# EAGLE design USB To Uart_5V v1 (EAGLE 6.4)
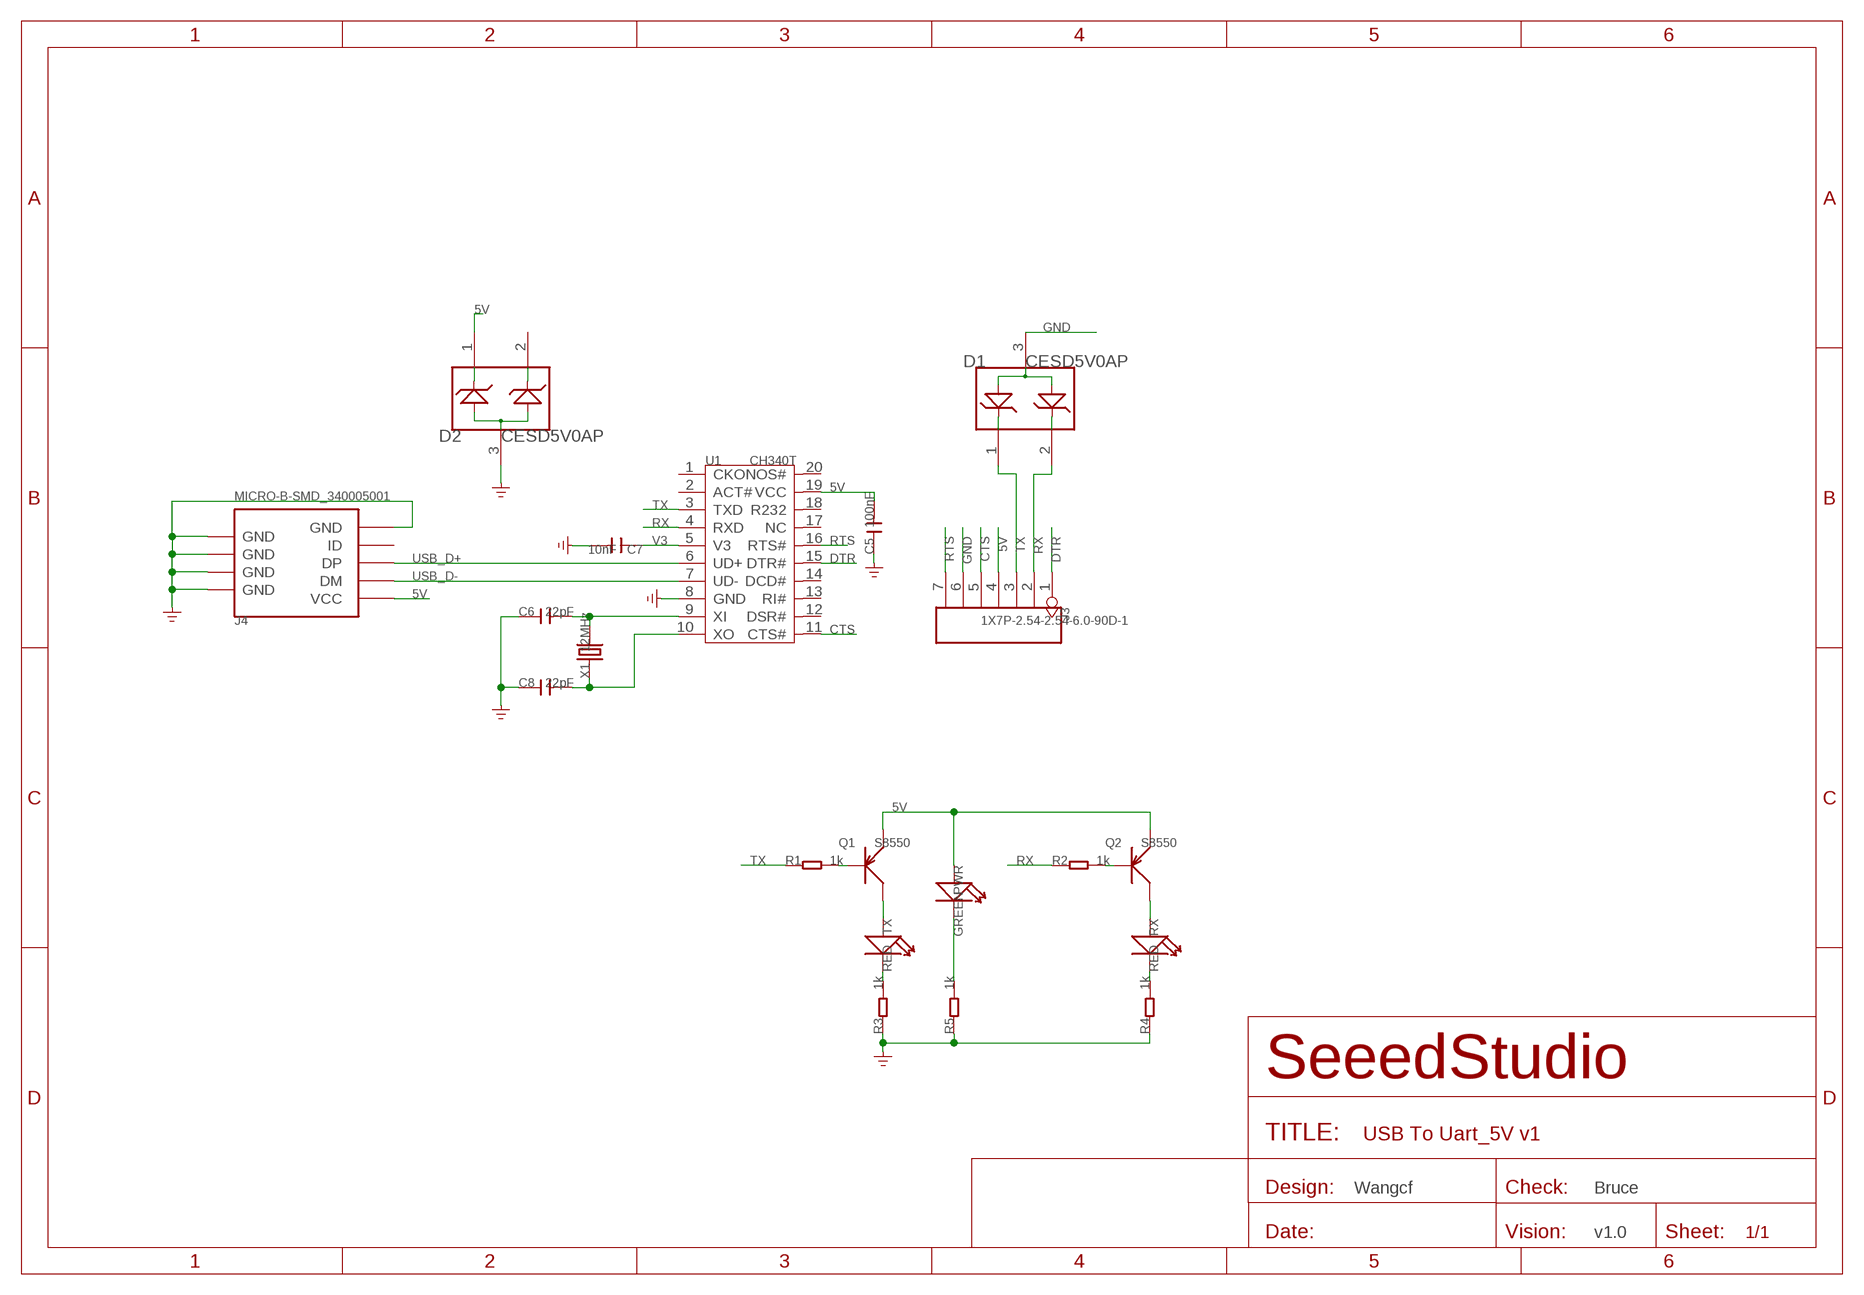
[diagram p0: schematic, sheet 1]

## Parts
C5  100nF  C-0402  [C0402]
C6  22pF  C-0402  [C0402]
C7  10nF  C-0402  [C0402]
C8  22pF  C-0402  [C0402]
D1  CESD5V0AP  D-ESD-3P  [SOT23]
D2  CESD5V0AP  D-ESD-3P  [SOT23]
J3  1X7P-2.54-2.54-6.0-90D-1  HEADER-7P  [7P-2.54-65/35MIL]
J4  MICRO-B-SMD_340005001  USB-MINIUSB-5P-MICRO  [MICRO-USB]
PWR  GREEN  LED'0603'  [LED-0603]
Q1  S8550  TRANSISTOR-PNP-SOT23  [SOT23]
Q2  S8550  TRANSISTOR-PNP-SOT23  [SOT23]
R1  1k  R-0402  [R0402]
R2  1k  R-0402  [R0402]
R3  1k  R-0402  [R0402]
R4  1k  R-0402  [R0402]
R5  1k  R-0402  [R0402]
RX  RED  LED'0603'  [LED-0603]
TX  RED  LED'0603'  [LED-0603]
U1  CH340T  [SSOP20]
X1  12MHz  CRYSTAL'HC49UP'  [HC49UP]

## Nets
5V: C5.2 D2.1 J3.4 J4.1(VCC) PWR.+ Q1.2(E) Q2.2(E) U1.19(VCC)
CTS: J3.5 U1.11(CTS#)
DTR: J3.1 U1.15(DTR#)
GND: C5.1 C6.1 C7.2 C8.1 D1.3 D2.3 J3.6 J4.5(GND) J4.S1(GND) J4.S2(GND) J4.S3(GND) J4.S4(GND) J4.S5(GND) J4.S6(GND) R3.1 R4.1 R5.1 U1.8(GND)
N$1: Q1.3(C) TX.+
N$2: Q2.3(C) RX.+
N$4: C6.2 U1.9(XI) X1.2
N$5: C8.2 U1.10(XO) X1.1
N$6: R3.2 TX.-
N$7: Q1.1(B) R1.2
N$8: Q2.1(B) R2.2
N$10: R4.2 RX.-
N$12: PWR.- R5.2
RTS: J3.7 U1.16(RTS#)
RX: D1.2 J3.2 R2.1 U1.4(RXD)
TX: D1.1 J3.3 R1.1 U1.3(TXD)
USB_D+: J4.3(DP) U1.6(UD+)
USB_D-: J4.2(DM) U1.7(UD-)
V3: C7.1 U1.5(V3)
Unconnected: D2.2 J4.4(ID) U1.1(CKO) U1.2(ACT#) U1.12(DSR#) U1.13(RI#) U1.14(DCD#) U1.17(NC) U1.18(R232) U1.20(NOS#)

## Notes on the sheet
- Wangcf | Bruce
- v1.0

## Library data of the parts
C5-C8 = Discrete:C*: Ceramic Capacitors
D1 D2 = Discrete:D-ESD-3P
J3 = Connector :HEADER-7P
J4 = Connector :USB-MINIUSB-5P
PWR RX TX = Discrete:LED*
Q1 Q2 = Discrete:TRANSISTOR-PNP*: PNP audion
R1-R5 = Discrete:R*
U1 = template:CH340T
X1 = Discrete:CRYSTAL*: CRYSTAL

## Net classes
0 default: width 0.152 mm, drill 0.305 mm, clearance 0.152 mm

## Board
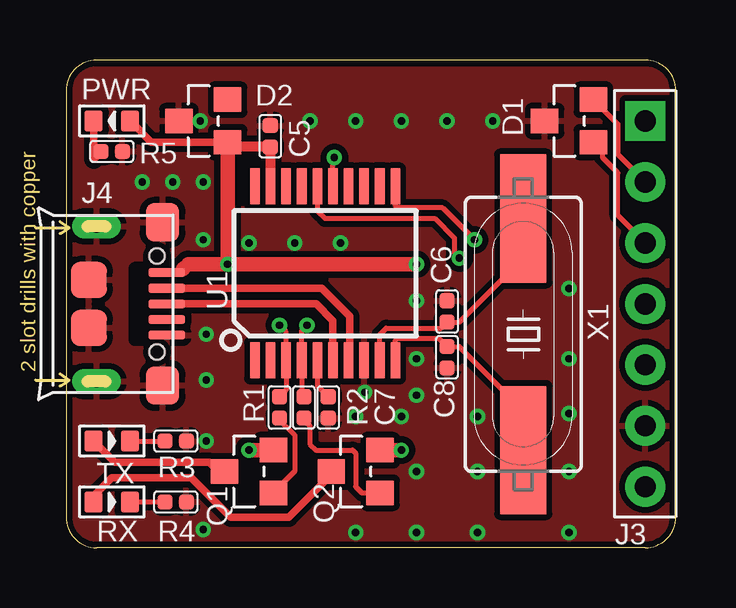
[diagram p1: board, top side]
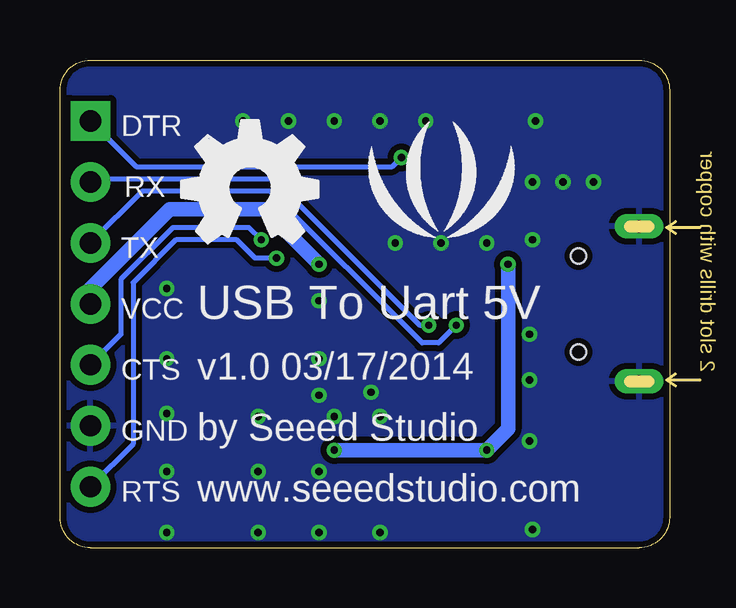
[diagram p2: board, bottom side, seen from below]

Size 25.4 x 20.32 mm. Coordinates in mm from the lower left corner, seen from the top.
Outline: 0,1.27 arc90 1.27,0
Outline: 24.13,0 arc90 25.4,1.27
Outline: 25.4,19.05 arc90 24.13,20.32
Outline: 1.27,20.32 arc90 0,19.05
Outline: 0,1.27 arc90 1.27,0
Outline: 24.13,0 arc90 25.4,1.27
Outline: 25.4,19.05 arc90 24.13,20.32
Outline: 1.27,20.32 arc90 0,19.05
Outline: 0,19.05 0,1.27
Outline: 0,1.27 arc90 1.27,0
Outline: 24.13,0 arc90 25.4,1.27
Outline: 25.4,1.27 25.4,19.05
Outline: 25.4,19.05 arc90 24.13,20.32
Outline: 24.13,20.32 1.27,20.32
Outline: 1.27,20.32 arc90 0,19.05
Outline: 24.13,0 1.27,0
Copper layers (1*16): Top 0.035mm / dielectric 1.5mm / Bottom 0.035mm
Design rules "SeeedStudio_2layer_DRU_no_angle_20140221 *": minimum track width 6mil, minimum drill 12mil, track to track 6mil, track to pad 6mil, pad to pad 6mil, via to via 6mil, smd to smd 0mil, copper to edge 10mil, drill to drill 10mil, minimum pad ring 10mil, minimum via ring 6mil, stop-mask expansion 2mil, vias tented up to drill 25mil, thermal gap 10mil

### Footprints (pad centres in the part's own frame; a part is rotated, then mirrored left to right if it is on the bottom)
C0402 = smd 0.635 x 0.635: 1 -0.445,0; 2 0.445,0
SOT23 = smd 1.016 x 1.143: 1 -0.889,-1.016; 2 0.889,-1.016; 3 0,1.016
7P-2.54-65/35MIL = drill 0.889 pad 1.651 square: 1 0,7.62 | drill 0.889 pad 1.651: 2 0,5.08; 3 0,2.54; 4 0,0; 5 0,-2.54; 6 0,-5.08; 7 0,-7.62
MICRO-USB = smd 0.381 x 1.524: 1 -1.3,-0.25; 2 -0.65,-0.25; 3 0,-0.25; 4 0.65,-0.25; 5 1.3,-0.25 | smd 1.6 x 1.397: S1 -3.4,-0.427; S6 3.4,-0.427 | drill 0.508 pad 1.016 long: S2 -3.226,-3.175; S5 3.226,-3.175 | smd 1.5 x 1.5: S3 -1,-3.5; S4 1,-3.5 | hole 0.635: -2,-0.65; 2,-0.65
LED-0603 = smd 0.762 x 0.889: + -0.762,0; - 0.762,0
R0402 = smd 0.635 x 0.635: 1 -0.445,0; 2 0.445,0
SSOP20 = smd 0.4 x 1.5: 1 -2.925,-3.625; 2 -2.275,-3.625; 3 -1.625,-3.625; 4 -0.975,-3.625; 5 -0.325,-3.625; 6 0.325,-3.625; 7 0.975,-3.625; 8 1.625,-3.625; 9 2.275,-3.625; 10 2.925,-3.625; 11 2.925,3.625; 12 2.275,3.625; 13 1.625,3.625; 14 0.975,3.625; 15 0.325,3.625; 16 -0.325,3.625; 17 -0.975,3.625; 18 -1.625,3.625; 19 -2.275,3.625; 20 -2.925,3.625
HC49UP = smd 5.334 x 1.93: 1 -4.826,0; 2 4.826,0

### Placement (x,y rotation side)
C5  8.51,17.14 270 top
C6  15.88,9.84 270 top
C7  10.92,5.84 270 top
C8  15.88,7.94 90 top
D1  20.95,17.78 90 top
D2  5.71,17.78 90 top
J3  24.13,10.16 0 top
J4  4.45,10.16 270 top
PWR  1.91,17.78 180 top
Q1  7.62,3.17 90 top
Q2  12.06,3.17 90 top
R1  8.89,5.84 270 top
R2  9.91,5.84 270 top
R3  4.57,4.45 180 top
R4  4.57,1.91 180 top
R5  1.91,16.51 180 top
RX  1.91,1.91 0 top
TX  1.91,4.45 0 top
U1  10.79,11.43 0 top
U$8  [LOGO_SILK]  9.53,14.61 0 bottom
U$9  [OSHW_FILLX200_NOTEXT]  20.32,12.7 0 bottom
X1  19.05,8.89 90 top

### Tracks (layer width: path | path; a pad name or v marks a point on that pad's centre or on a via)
5V  (via drill 0.3 pad 0.64)
  Top 0.305: D2.1 3.56,16.89 PWR.+ | J4.1 4.73,11.46 4.89,11.62
  Top 0.406: PWR.+ 2.67,17.65 | D2.1 6.92,16.7 C5.2 U1.19
  Top 0.61: v6.73,11.81 D2.1 | v7.62,4.06 Q1.2 | v13.97,4.06 Q2.2 | 4.89,11.62 5.08,11.81 v6.73,11.81 | v6.73,11.81 v14.61,11.81
  Bottom 0.61: v6.73,11.81 6.73,4.95 v7.62,4.06 v13.97,4.06 | v14.61,11.81 16.89,14.1 20.83,14.1 24.13,10.79 J3.4
CTS  (via drill 0.3 pad 0.64)
  Top 0.203: v17.02,12.83 15.68,14.16 13.81,14.16 13.72,14.25 U1.11
  Bottom 0.203: v17.02,12.83 17.53,13.34 20.7,13.34 22.86,11.18 22.86,8.89 J3.5
DTR  (via drill 0.3 pad 0.64)
  Top 0.203: U1.15 11.12,16.2 v11.18,16.26
  Bottom 0.203: v11.18,16.26 11.56,15.88 22.23,15.88 J3.1
GND  (via drill 0.3 pad 0.64)
  other vias: 5.71,0.76 9.53,12.7 7.62,12.7 4.45,15.24 3.17,15.24 11.43,12.7 12.06,5.46 12.45,6.48 13.97,5.46 14.61,6.35 14.61,7.87 5.84,4.45 5.84,6.99 5.84,8.89 12.06,0.64 17.14,0.64 17.78,17.78 12.06,17.78 15.88,17.78 10.16,17.78 5.59,17.78 5.71,15.24 5.71,12.83 13.97,17.78 14.61,3.17 14.61,0.64 17.14,3.17 17.14,5.46 20.95,0.64 20.95,3.17 20.95,5.59 20.95,7.87 20.95,10.79 14.61,10.29
  pour Top (isolate 0.254): 0,20.32 25.4,20.32 25.4,0 0,0
  pour Bottom (isolate 0.254): 0,20.32 25.4,20.32 25.4,0 0,0
N$1
  Top 0.305: Q1.3 6.35,3.17 5.97,3.56 2.03,3.56 TX.+
N$2
  Top 0.305: RX.+ 1.14,2.16 1.91,2.92 5.21,2.92 6.86,1.27 9.28,1.27 11.05,3.04 Q2.3
N$4
  Top 0.203: U1.9 13.07,8.88 13.34,9.14 15.62,9.14 C6.2 16.38,9.4 18.41,11.43 18.41,13.08 X1.2
N$5
  Top 0.203: U1.10 13.72,8.64 13.81,8.73 15.52,8.73 C8.2 16.38,8.38 19.05,5.71 X1.1 19.05,3.81 19.05,3.56
N$6
  Top 0.203: TX.- R3.2
N$7
  Top 0.203: R1.2 8.89,5.33 9.53,4.7 9.53,3.17 Q1.1
N$8
  Top 0.203: R2.2 9.91,5.33 10.16,5.08 10.16,4.32 10.41,4.06 11.94,4.06 12.06,3.94 12.06,2.54 12.32,2.29 Q2.1
N$10
  Top 0.203: RX.- R4.2
N$12
  Top 0.305: PWR.- 1.14,16.19 R5.2
RTS  (via drill 0.3 pad 0.64)
  Top 0.203: U1.16 10.47,14.04 10.79,13.72 15.36,13.72 16.18,12.9 16.18,12.27 v16.38,12.06
  Bottom 0.203: v16.38,12.06 17.27,12.06 18.03,12.83 20.57,12.83 22.35,11.05 22.35,4.32 J3.7
RX  (via drill 0.3 pad 0.64)
  Top 0.203: R2.1 9.82,6.37 U1.4 9.82,9.06 v10.03,9.27 | D1.2 22.99,17.65 22.99,16.38 J3.2
  Bottom 0.203: v10.03,9.27 10.41,9.27 16.51,15.37 24,15.37 J3.2
TX  (via drill 0.3 pad 0.64)
  Top 0.203: R1.1 9.17,6.57 U1.3 9.17,8.99 v8.89,9.27 | D1.1 22.35,16.89 22.35,16.26 22.99,15.62 22.99,13.84 J3.3
  Bottom 0.203: v8.89,9.27 9.63,8.53 10.31,8.53 16.64,14.86 21.97,14.86 J3.3
USB_D+
  Top 0.305: U1.6 11.12,9.45 10.41,10.16 J4.3
USB_D-
  Top 0.305: J4.2 10.65,10.81 11.81,9.65 11.81,7.85 U1.7
V3
  Top 0.203: U1.5 10.47,6.74 C7.1

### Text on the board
bPlace: DTR | RX | TX | USB To Uart 5V | VCC | v1.0 03/17/2014 | CTS | by Seeed Studio | GND | www.seeedstudio.com | RTS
